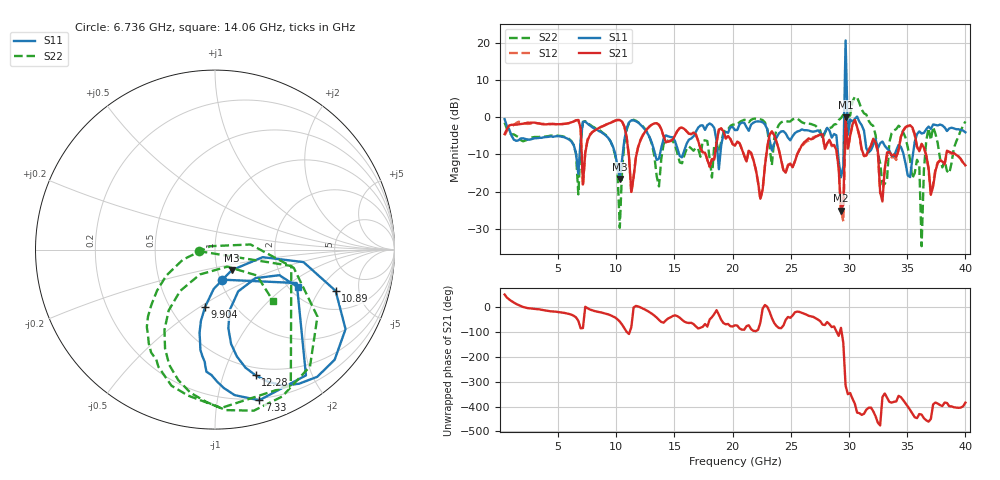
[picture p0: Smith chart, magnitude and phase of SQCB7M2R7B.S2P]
! Network Analyzer HP8722ES.07.66: Jul 25, 2000 Serial No. US39175408
! 26 Oct 2004  13:19:12
! Frequency  S11  S21  S12  S22
# HZ  S  DB R  50
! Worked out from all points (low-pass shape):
!   201 points, 400 MHz to 40 GHz, reference 50 ohm
!   highest |S21| = -0.03 dB at 29.7 GHz (marker M1); lowest = -25.1 dB at 29.31 GHz (marker M2)
!   |S21| within 3 dB of the highest: 641.3 MHz to 6.935 GHz (6.294 GHz wide, 166 % of centre); 8.434 GHz to 10.73 GHz (2.295 GHz wide, 24 % of centre)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
!   lowest |S11| = -16.6 dB at 10.3 GHz (marker M3), VSWR 1.35, Z = 58.5 - j13.7 ohm
!   |S11| at or under -10 dB: 9.916 GHz to 10.55 GHz (634.3 MHz wide, 6.2 % of centre); 29.06 GHz to 29.53 GHz (463.5 MHz wide, 1.58 % of centre); 34.68 GHz to 35.49 GHz (809.7 MHz wide, 2.31 % of centre)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
!   |S22| runs from -34.7 to 5.5 dB; largest |S21 - S12| = 0.66
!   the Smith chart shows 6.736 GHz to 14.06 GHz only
!   S11 on the Smith chart (normalised r, x): 6.736 GHz: 1.02, -0.35; 7.33 GHz: 0.18, -1.32; 9.904 GHz: 0.74, -0.52; 10.89 GHz: 3.09, -2.87; 12.28 GHz: 0.42, -1.29; 14.06 GHz: 2.23, -1.28
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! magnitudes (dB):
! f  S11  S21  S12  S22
! 400 MHz  -0.5  -4.5  -4.8  -1.5
! 6.736 GHz  -15.3  -0.8  -0.7  -20.7
! 7.132 GHz  -1.3  -18.1  -18.6  -1.2
! 7.33 GHz  -1.2  -9.6  -9.3  -1.1
! 9.904 GHz  -9.8  -0.9  -0.9  -10.2
! 10.3 GHz  -16.6  -0.8  -0.7  -29.7
! 10.89 GHz  -3.0  -5.5  -5.5  -3.3
! 12.28 GHz  -2.7  -4.9  -4.8  -2.4
! 13.67 GHz  -11.2  -2.1  -2.1  -18.6
! 14.06 GHz  -5.8  -5.1  -5.2  -7.3
! 20.2 GHz  -3.5  -7.6  -7.5  -2.0
! 22.38 GHz  -1.2  -21.9  -22.2  -0.6
! 26.93 GHz  -3.9  -5.7  -5.4  -2.1
! 29.31 GHz  -16.2  -25.1  -24.9  -0.2
! 29.51 GHz  -13.3  -23.5  -28.0  0.7
! 29.7 GHz  20.6  0.0  -3.2  -1.9
! 29.9 GHz  -4.8  -8.4  -8.8  -0.1
! 33.47 GHz  -9.0  -9.3  -10.0  -6.7
! 36.04 GHz  -3.8  -9.2  -9.2  -13.1
! 36.24 GHz  -4.4  -7.2  -7.2  -34.7
! 36.83 GHz  -2.5  -13.5  -14.1  -2.9
! 40 GHz  -4.1  -12.9  -13.1  -1.1
